PROGRAM MAIN
VAR
	ENABLE:BOOL;

//RECIPE
PROCESS:PROCESS;
PROCESS_EN:BOOL;
PROCESS_RUN:BOOL;
PROCESS_STOP:BOOL;

P_NO:INT;

CYCLE_EN:BOOL;
CYCLE_NUM:INT;
CYCLE_START_STEP_NO:INT;

STEP_NO:INT;
NEXTSTEP_EN:BOOL;

UPS:FB_S_UPS_BAPI;

END_VAR

//UPS
UPS(
	sNetID:= , 
	iPLCPort:= 851, 
	tTimeout:= , 
	eUpsMode:= eSUPS_WrPersistData_shutdown, 
	ePersistentMode:= , 
	tRecoverTime:= T#10S, 
	bPowerFailDetect=> , 
	eState=> , 
	nCapacity=> , 
	bBusy=> , 
	bError=> , 
	nErrID=> );

//******************************IO*********************************
	IO_EXCHANGE();

//*****************************CONFIGURATION***********************
	IL();

//*****************************INTERLOCK***************************
	Temp();
	
//*****************************PROCESS*****************************
	PROCESS_RUN:=GV.Process_Start AND NOT GV.ALARM_OCC;
	PROCESS_STOP:=GV.Process_Stop OR GV.ALARM_OCC;

	//PROCESS ENABLE
	IF PROCESS_RUN AND NOT PROCESS_EN
		THEN
		CYCLE_NUM := 0;
		STEP_NO:=1;
		P_NO:=1;
		PM.ProcessFeedBack.ProcessFinished:=FALSE;
	END_IF
		IF PROCESS_RUN AND NOT PROCESS_EN
		THEN
		PROCESS_EN:=TRUE;		
	END_IF;
	
	IF PROCESS_STOP
		THEN
		CYCLE_NUM:=0;
		CYCLE_EN:=FALSE;
		PROCESS_EN:=FALSE;
		PROCESS_RUN:=FALSE;
	END_IF;
	IF NOT PM.ProcessFeedBack.ProcessFinished
		THEN 
			PM.ProcessFeedBack.CurrentStepNo:=STEP_NO;
		ELSE
			PM.ProcessFeedBack.CurrentStepNo:=STEP_NO-1;
	END_IF
	
	IF PROCESS_EN
		THEN 
		PM.ProcessFeedBack.ProcessStart:=TRUE;
		PM.ProcessFeedBack.CurrentStepstart:=TRUE;
		ELSE
			PM.ProcessFeedBack.ProcessStart:=FALSE;
			PM.ProcessFeedBack.CurrentStepstart:=FALSE;
		END_IF
	
	IF GV.Step_Num<STEP_NO 
		THEN 	
		PM.ProcessFeedBack.ProcessFinished:=TRUE;
	END_IF
	IF  GV.ALARM_OCC
		THEN
		PROCESS_EN:=FALSE;	
		
	END_IF
	
	IF STEP_NO<1 OR STEP_NO >100
		THEN 
		STEP_NO:=1;
	END_IF
	
	//CYCLE初始化
	IF GV.SetpArray[STEP_NO].CycleStart AND CYCLE_EN=FALSE
		THEN 
		CYCLE_EN				:=	TRUE;
		CYCLE_START_STEP_NO		:=	STEP_NO;
		CYCLE_NUM				:=	GV.SetpArray[STEP_NO].CycleNumber;
	END_IF;	
	
	//STEP
	PROCESS(
	ENABLE			:= 	PROCESS_EN, 
	NEXTSTEP_EN		:=	NEXTSTEP_EN,
	Alarm_RST		:=	UI.Warning_And_Alarm_RST,
	PMStableTime	:=	GV.PMConfig.PMStableTime,
	STEP_DATA		:= 	GV.SetpArray[STEP_NO],  
	);
	
	//PROCESS FLOW	
	CASE P_NO OF
		1:	IF NOT PROCESS_EN 
				THEN 
				P_NO:=100;
				ELSE
				P_NO:=2;	
			END_IF;
			NEXTSTEP_EN:=FALSE;
			
		2:	IF PROCESS.NEXTSTEP 
				THEN 
				PM.ProcessFeedBack.CurrentStepFinished:=TRUE;
				PM.ProcessFeedBack.CurrentStepstart:=FALSE;
				P_NO:=3;
			END_IF;
			
		3:	IF CYCLE_EN
			THEN
				P_NO:=10;
				ELSE
				P_NO:=20;
			END_IF
		
		10:	IF GV.SetpArray[STEP_NO].CycleEnd 
				THEN 
				P_NO:=11; 
				ELSE
				P_NO:=20; 
			END_IF;	
		
		11:	IF CYCLE_NUM=0 
				THEN 
				P_NO:=20; 
				CYCLE_EN:=FALSE;
				ELSE
				CYCLE_NUM:=CYCLE_NUM-1; 
				P_NO:=21; 
			END_IF;	
				
		20:	STEP_NO:=STEP_NO+1;
			NEXTSTEP_EN:=TRUE;
			P_NO:=1; 
			PM.ProcessFeedBack.CurrentStepstart:=TRUE;
			PM.ProcessFeedBack.CurrentStepFinished:=FALSE;
			
		21:	STEP_NO:=CYCLE_START_STEP_NO;
			NEXTSTEP_EN:=TRUE;
			P_NO:=1;
		
		100:;	
	END_CASE;	
		
	
	IF	PROCESS_EN
		THEN
//******************工艺参数赋值***************
		//APC
		GV.	AO.	APC.TARGET_PRESSURE	:=	PROCESS.APC_PRESSURE;
		GV.	AO.	APC.TARGET_POSITION	:=	PROCESS.APC_POSITION;
		IF GV_IL.APC_EN THEN 
		GV.AO.	APC.	Control_Mode	:=	PROCESS.APC_CONTROL_MODE	;
		ELSE 
		GV.AO.	APC.	Control_Mode	:=	3	;
		END_IF
		
		//MFC
		GV.AO.MFC1_Flow_Setpoint	:=	PROCESS.MFC1_SV;
		GV.AO.MFC2_Flow_Setpoint	:=	PROCESS.MFC2_SV;
		GV.AO.MFC3_Flow_Setpoint	:=	PROCESS.MFC3_SV;
		GV.AO.MFC4_Flow_Setpoint	:=	PROCESS.MFC4_SV;
		GV.AO.MFC5_Flow_Setpoint	:=	PROCESS.MFC5_SV;
		GV.AO.MFC6_Flow_Setpoint	:=	PROCESS.MFC6_SV;
		GV.AO.MFC7_Flow_Setpoint	:=	PROCESS.MFC7_SV;
	//	GV.AO.MFC8_Flow_Setpoint	:=	PROCESS.MFC8_SV;
	//	GV.AO.MFC9_Flow_Setpoint	:=	PROCESS.MFC9_SV;
		
//LID HEATER
		GV.AO.LID_Temp_SV			:=	PROCESS.LID_TEMP;		
		
//CHAMBER HEATER
		GV.AO.	Chamber_Temp1_SV	:=	
		GV.AO.	Chamber_Temp2_SV	:=	
		GV.AO.	Chamber_Temp3_SV	:=	PROCESS.WALL_TEMP;
//STAGE
		GV.AO.Stage_Temp1_SV	 	:=	PROCESS.STAGE_TEMP1;
		GV.AO.Stage_Temp1_SV	 	:=	PROCESS.STAGE_TEMP2;	
		GV.AO.Stage_Temp1_SV	 	:=	PROCESS.STAGE_TEMP3;	
		GV.AO.Stage_Temp1_SV	 	:=	PROCESS.STAGE_TEMP4;		
		
//************************TOLERANCE 赋值****************
		

//************************VALVE动作****************
		GV.NDO.AV1	:=	FALSE	;//	(	GV.AO.MFC1_Flow_Setpoint>0	)	AND	PM.INFO.Alarm.TOLERANCE_MFC1	AND	GV_IL.AV1_EN	;
		GV.NDO.AV2	:=			(	GV.AO.MFC1_Flow_Setpoint>0	)	AND	PM.INFO.Alarm.TOLERANCE_MFC1	AND	GV_IL.AV2_EN	;
		GV.NDO.AV3	:=	FALSE	;//(	GV.AO.MFC1_Flow_Setpoint>0	)	AND	PM.INFO.Alarm.TOLERANCE_MFC1	AND	GV_IL.AV3_EN	;
		GV.NDO.AV4	:=	FALSE	;//	(	GV.AO.MFC2_Flow_Setpoint>0	)	AND	PM.INFO.Alarm.TOLERANCE_MFC2	AND	GV_IL.AV4_EN	;
		GV.NDO.AV5	:=			(	GV.AO.MFC1_Flow_Setpoint>0	)	AND	PM.INFO.Alarm.TOLERANCE_MFC1	AND	GV_IL.AV5_EN	;
		GV.NDO.AV6	:=	FALSE	;//	(	GV.AO.MFC2_Flow_Setpoint>0	)	AND	PM.INFO.Alarm.TOLERANCE_MFC2	AND	GV_IL.AV6_EN	;
		GV.NDO.AV7	:=	FALSE	;//	(	GV.AO.MFC3_Flow_Setpoint>0	)	AND	PM.INFO.Alarm.TOLERANCE_MFC3	AND	GV_IL.AV7_EN	;
		GV.NDO.AV8	:=	FALSE	;//	(	GV.AO.MFC3_Flow_Setpoint>0	)	AND	PM.INFO.Alarm.TOLERANCE_MFC3	AND	GV_IL.AV8_EN	;
		GV.NDO.AV9	:=	FALSE	;//	(	GV.AO.MFC3_Flow_Setpoint>0	)	AND	PM.INFO.Alarm.TOLERANCE_MFC3	AND	GV_IL.AV9_EN	;
		GV.NDO.AV10	:=	FALSE	;//	(		)	AND		AND	GV_IL.AV10_EN	;
		GV.NDO.AV11	:=	FALSE	;//	(		)	AND		AND	GV_IL.AV11_EN	;
		GV.NDO.AV12	:=	FALSE	;//	(		)	AND		AND	GV_IL.AV12_EN	;
		GV.NDO.AV13	:=	FALSE	;//	(		)	AND		AND	GV_IL.AV13_EN	;
		GV.NDO.AV14	:=	FALSE	;//	(	GV.AO.MFC5_Flow_Setpoint>0	)	AND	PM.INFO.Alarm.TOLERANCE_MFC5	AND	GV_IL.AV14_EN	;
		GV.NDO.AV15	:=	FALSE	;//	(	GV.AO.MFC5_Flow_Setpoint>0	)	AND	PM.INFO.Alarm.TOLERANCE_MFC5	AND	GV_IL.AV15_EN	;
		GV.NDO.AV16	:=	FALSE	;//	(	GV.AO.MFC5_Flow_Setpoint>0	)	AND	PM.INFO.Alarm.TOLERANCE_MFC5	AND	GV_IL.AV16_EN	;
		GV.NDO.AV17	:=	FALSE	;//	(		)	AND		AND	GV_IL.AV17_EN	;
		GV.NDO.AV18	:=	FALSE	;//	(		)	AND		AND	GV_IL.AV18_EN	;
		GV.NDO.AV19	:=	FALSE	;//	(		)	AND		AND	GV_IL.AV19_EN	;
		GV.NDO.AV20	:=	FALSE	;//	(	GV.AO.MFC6_Flow_Setpoint>0	)	AND	PM.INFO.Alarm.TOLERANCE_MFC6	AND	GV_IL.AV20_EN	;
		GV.NDO.AV21	:=	FALSE	;//	(	GV.AO.MFC6_Flow_Setpoint>0	)	AND	PM.INFO.Alarm.TOLERANCE_MFC6	AND	GV_IL.AV21_EN	;
		GV.NDO.AV22	:=	FALSE	;//	(	GV.AO.MFC6_Flow_Setpoint>0	)	AND	PM.INFO.Alarm.TOLERANCE_MFC6	AND	GV_IL.AV22_EN	;
		GV.NDO.AV23	:=	FALSE	;//	(	GV.AO.MFC7_Flow_Setpoint>0	)	AND	PM.INFO.Alarm.TOLERANCE_MFC7	AND	GV_IL.AV23_EN	;
		GV.NDO.AV24	:=	FALSE	;//	(	GV.AO.MFC7_Flow_Setpoint>0	)	AND	PM.INFO.Alarm.TOLERANCE_MFC7	AND	GV_IL.AV24_EN	;
		GV.NDO.AV25	:=	FALSE	;//	(	GV.AO.MFC7_Flow_Setpoint>0	)	AND	PM.INFO.Alarm.TOLERANCE_MFC7	AND	GV_IL.AV25_EN	;
		GV.NDO.AV26	:=			(	GV.AO.MFC1_Flow_Setpoint>0	)	AND	PM.INFO.Alarm.TOLERANCE_MFC1	AND	GV_IL.AV26_EN	;
							(*	(
						((	GV.AO.MFC1_Flow_Setpoint>0	)	AND	PM.INFO.Alarm.TOLERANCE_MFC1) 
					OR ((	GV.AO.MFC2_Flow_Setpoint>0	)	AND	PM.INFO.Alarm.TOLERANCE_MFC2)
					OR ((	GV.AO.MFC3_Flow_Setpoint>0	)	AND	PM.INFO.Alarm.TOLERANCE_MFC3)
						)
						AND	GV_IL.AV26_EN	;*)
		GV.NDO.AV27	:=	FALSE	;(*	(	
						((	GV.AO.MFC5_Flow_Setpoint>0	)	AND	PM.INFO.Alarm.TOLERANCE_MFC5)
					OR 	((	GV.AO.MFC6_Flow_Setpoint>0	)	AND	PM.INFO.Alarm.TOLERANCE_MFC6)
					OR	((	GV.AO.MFC7_Flow_Setpoint>0	)	AND	PM.INFO.Alarm.TOLERANCE_MFC7)	
						)	
						AND	GV_IL.AV27_EN	;*)

		
	END_IF

//TOL ALRM&WARNING
	PM.INFO.Alarm.TOLERANCE_PRESSURE			:= NOT PROCESS.PRESSURE_ALARM;
	PM.INFO.Alarm.TOLERANCE_MFC1				:= NOT PROCESS.MFC1_Alarm;
	PM.INFO.Alarm.TOLERANCE_MFC2				:= NOT PROCESS.MFC2_Alarm;
	PM.INFO.Alarm.TOLERANCE_MFC3				:= NOT PROCESS.MFC3_Alarm;
	PM.INFO.Alarm.TOLERANCE_MFC4				:= NOT PROCESS.MFC4_Alarm;
	PM.INFO.Alarm.TOLERANCE_MFC5				:= NOT PROCESS.MFC5_Alarm;
	PM.INFO.Alarm.TOLERANCE_MFC6				:= NOT PROCESS.MFC6_Alarm;
	PM.INFO.Alarm.TOLERANCE_MFC7				:= NOT PROCESS.MFC7_Alarm;
	PM.INFO.Alarm.TOLERANCE_MFC8				:= NOT PROCESS.MFC8_Alarm;
	PM.INFO.Alarm.TOLERANCE_MFC9				:= NOT PROCESS.MFC9_Alarm;
	PM.INFO.Alarm.TOLERANCE_WALL_TEMP			:= NOT PROCESS.WALL_TEMP_Alarm;
	PM.INFO.Alarm.TOLERANCE_LID_TEMP			:= NOT PROCESS.LID_TEMP_Alarm;
	PM.INFO.Alarm.TOLERANCE_STAGE_TEMP1			:= NOT PROCESS.STAGE_TEMP1_Alarm;
	PM.INFO.Alarm.TOLERANCE_STAGE_TEMP2			:= NOT PROCESS.STAGE_TEMP2_Alarm;
	PM.INFO.Alarm.TOLERANCE_STAGE_TEMP3			:= NOT PROCESS.STAGE_TEMP3_Alarm;
	PM.INFO.Alarm.TOLERANCE_STAGE_TEMP4			:= NOT PROCESS.STAGE_TEMP4_Alarm;
	
	PM.INFO.Warning.TOLERANCE_PRESSURE			:= NOT PROCESS.PRESSURE_WARNING;	
	PM.INFO.Warning.TOLERANCE_MFC1				:= NOT PROCESS.MFC1_WARNING;
	PM.INFO.Warning.TOLERANCE_MFC2				:= NOT PROCESS.MFC2_WARNING;
	PM.INFO.Warning.TOLERANCE_MFC3				:= NOT PROCESS.MFC3_WARNING;
	PM.INFO.Warning.TOLERANCE_MFC4				:= NOT PROCESS.MFC4_WARNING;
	PM.INFO.Warning.TOLERANCE_MFC5				:= NOT PROCESS.MFC5_WARNING;
	PM.INFO.Warning.TOLERANCE_MFC6				:= NOT PROCESS.MFC6_WARNING;
	PM.INFO.Warning.TOLERANCE_MFC7				:= NOT PROCESS.MFC7_WARNING;
	PM.INFO.Warning.TOLERANCE_MFC8				:= NOT PROCESS.MFC8_WARNING;
	PM.INFO.Warning.TOLERANCE_MFC9				:= NOT PROCESS.MFC9_WARNING;
	PM.INFO.Warning.TOLERANCE_WALL_TEMP			:= NOT PROCESS.WALL_TEMP_WARNING;	
	PM.INFO.Warning.TOLERANCE_LID_TEMP			:= NOT PROCESS.LID_TEMP_WARNING;	
	PM.INFO.Warning.TOLERANCE_STAGE_TEMP1		:= NOT PROCESS.STAGE_TEMP1_WARNING;		
	PM.INFO.Warning.TOLERANCE_STAGE_TEMP2		:= NOT PROCESS.STAGE_TEMP2_WARNING;	
	PM.INFO.Warning.TOLERANCE_STAGE_TEMP3		:= NOT PROCESS.STAGE_TEMP3_WARNING;		
	PM.INFO.Warning.TOLERANCE_STAGE_TEMP4		:= NOT PROCESS.STAGE_TEMP4_WARNING;

END_PROGRAM
